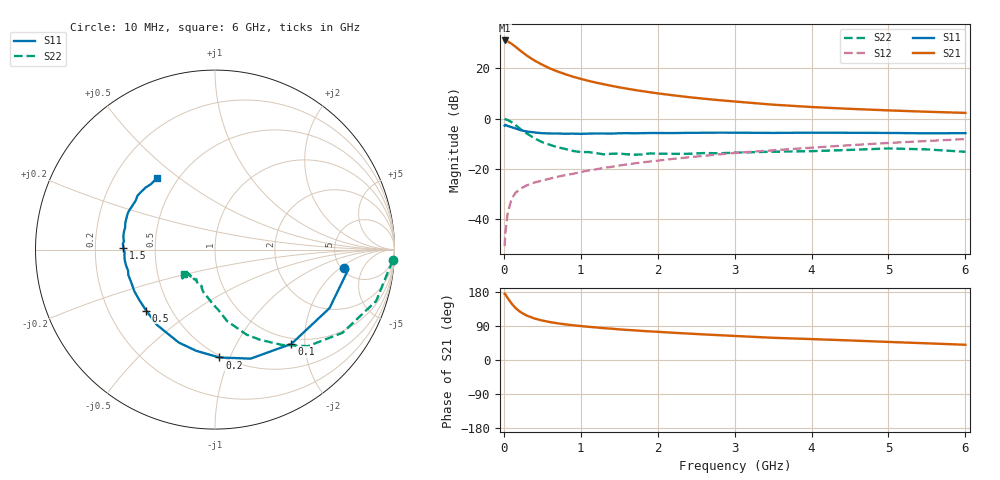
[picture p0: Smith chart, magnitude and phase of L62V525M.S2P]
!  INFINEON TECHNOLOGIES Small Signal Semiconductors
! BFR380L3 , Si-NPN RF-Transistor in TSLP-3-1
!  Vce=2.5 V,  Ic=25 mA
! Common Emitter S-Parameters:  07. March 2005
#  GHz  S  MA  R  50
! f  S11  S21  S12  S22
! GHz  Mag  Ang  Mag  Ang  Mag  Ang  Mag  Ang
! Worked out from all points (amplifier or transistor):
!   36 points, 10 MHz to 6 GHz, reference 50 ohm
!   highest |S21| = 31.1 dB at 10 MHz (marker M1)
!   |S21| within 3 dB of that: start of sweep to 171.5 MHz
!   unconditionally stable (mu >= 1): 1.856 GHz to 4.821 GHz
!   at 250 MHz: K = 0.40, MSG = 26.8 dB, |S12| = -27.3 dB
!   at 1.4 GHz: K = 0.96, MSG = 16.1 dB, |S12| = -19.2 dB
!   at 6 GHz: K = 0.98, MSG = 5.2 dB, |S12| = -8.1 dB
!   S11 on the Smith chart (normalised r, x): 10 MHz: 5.32, -2.24; 100 MHz: 0.90, -1.73; 200 MHz: 0.49, -0.92; 500 MHz: 0.36, -0.33; 1.5 GHz: 0.32, +0.01; 6 GHz: 0.39, +0.42
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0.01  0.7259 -7.9  35.91 174.7  0.0029 82.5  0.9922 -3.5
0.02  0.7512 -8.4  35.71 173.3  0.0054 95.3  0.9717 -7.3
0.05  0.7165 -27.1  34.4 163.3  0.0132 79.2  0.943 -17.6
0.1  0.6761 -51.0  30.9 149.2  0.0251 68.1  0.8484 -33.1
0.15  0.6392 -71.9  27.05 137.6  0.0332 61.1  0.7467 -46.1
0.2  0.6014 -87.7  23.41 129.0  0.0387 57.5  0.6503 -54.8
0.25  0.5735 -100.6  20.45 122.4  0.0431 53.9  0.5629 -63.3
0.3  0.5556 -111.4  17.9 117.1  0.0472 52.5  0.505 -69.7
0.4  0.5298 -127.5  14.28 109.4  0.0537 51.7  0.4037 -80.4
0.5  0.5125 -138.5  11.8 104.2  0.0587 52.1  0.34 -86.4
0.6  0.5066 -146.9  9.96 100.0  0.0641 53.3  0.3005 -92.8
0.8  0.5012 -158.6  7.642 94.0  0.0754 56.0  0.2491 -104.6
0.9  0.5032 -163.7  6.816 91.7  0.0798 57.7  0.2275 -108.9
1.1  0.5036 -170.1  5.65 87.6  0.0928 59.8  0.2161 -114.7
1.5  0.5104 179.1  4.199 80.8  0.1165 62.1  0.2021 -125.1
1.8  0.5142 172.8  3.524 76.7  0.1347 63.1  0.1941 -130.5
2.2  0.5157 166.2  2.912 71.9  0.1582 63.6  0.199 -133.7
2.8  0.5266 157.3  2.329 65.5  0.1942 63.9  0.2046 -140.0
3.5  0.5194 148.5  1.895 58.6  0.2343 62.4  0.22 -139.2
4.5  0.5226 142.2  1.565 51.6  0.296 61.1  0.2386 -138.9
5.5  0.5099 134.1  1.371 44.0  0.3589 57.6  0.2443 -138.6
6  0.5142 128.9  1.3 40.2  0.392 55.5  0.2187 -141.0
